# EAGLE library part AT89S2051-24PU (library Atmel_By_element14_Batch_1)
Microcontroller
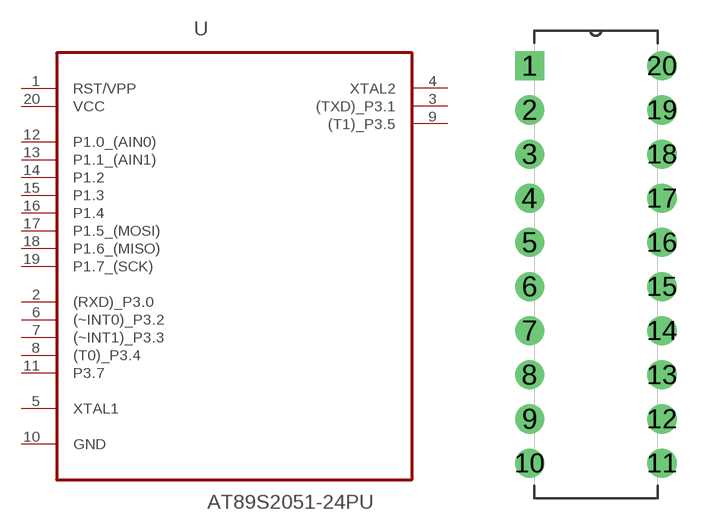
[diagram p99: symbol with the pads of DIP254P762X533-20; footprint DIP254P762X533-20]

Designator prefix U

## AT89S2051-24PU (DESCRIPTION: Microcontroller; MPN: AT89S2051-24PU; OC_FARNELL: 1095734; OC_NEWARK: 96K6573; PACKAGE: PDIP-20; SUPPLIER: ATMEL)  [DIP254P762X533-20]
1  RST/VPP  pwr
2  (RXD)_P3.0  in
3  (TXD)_P3.1  out
4  XTAL2  out
5  XTAL1  in
6  (~INT0)_P3.2
7  (~INT1)_P3.3
8  (T0)_P3.4  in
9  (T1)_P3.5  out
10  GND  pas
11  P3.7
12  P1.0_(AIN0)
13  P1.1_(AIN1)
14  P1.2
15  P1.3
16  P1.4
17  P1.5_(MOSI)
18  P1.6_(MISO)
19  P1.7_(SCK)  in
20  VCC  pwr

## Footprint DIP254P762X533-20 (pad centres in mm)
drill 1.118 square: 1 -7.62,22.86
drill 1.118: 2 -7.62,20.32; 3 -7.62,17.78; 4 -7.62,15.24; 5 -7.62,12.7; 6 -7.62,10.16; 7 -7.62,7.62; 8 -7.62,5.08; 9 -7.62,2.54; 10 -7.62,0; 11 0,0; 12 0,2.54; 13 0,5.08; 14 0,7.62; 15 0,10.16; 16 0,12.7; 17 0,15.24; 18 0,17.78; 19 0,20.32; 20 0,22.86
